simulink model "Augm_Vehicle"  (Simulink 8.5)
settings: Solver=ode45  StartTime=0.0  StopTime=10.0  RelTol=1e-3
undefined symbols (not defined in the file or in its folder): Al, Bl, Cl, Dl

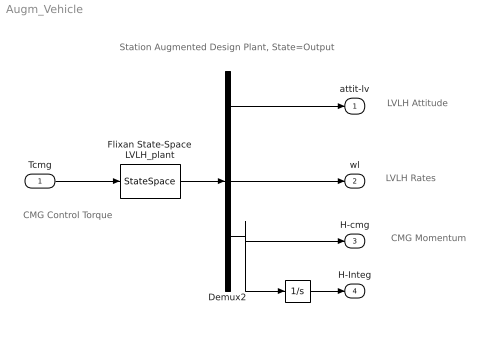
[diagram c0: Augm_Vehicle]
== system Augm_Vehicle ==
  note: LVLH Attitude
  note: LVLH Rates
  note: CMG Control Torque
  note: CMG Momentum
  note: Station Augmented Design Plant, State=Output
  Tcmg : Inport  PortDimensions=3
  "  " : Integrator
  Demux2 : Demux  Outputs=[3, 3, 3]
  Flixan State-Space LVLH_plant : StateSpace  A=Al  B=Bl  C=Cl  D=Dl  X0=0
  attit-lv : Outport
  wl : Outport  Port=2
  H-cmg : Outport  Port=3
  H-Integ : Outport  Port=4
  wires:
  Demux2/1 -> attit-lv/1
  Flixan State-Space LVLH_plant/1 -> Demux2/1
  Demux2/2 -> wl/1
  Demux2/3 -> "  "/1, H-cmg/1
  "  "/1 -> H-Integ/1
  Tcmg/1 -> Flixan State-Space LVLH_plant/1
